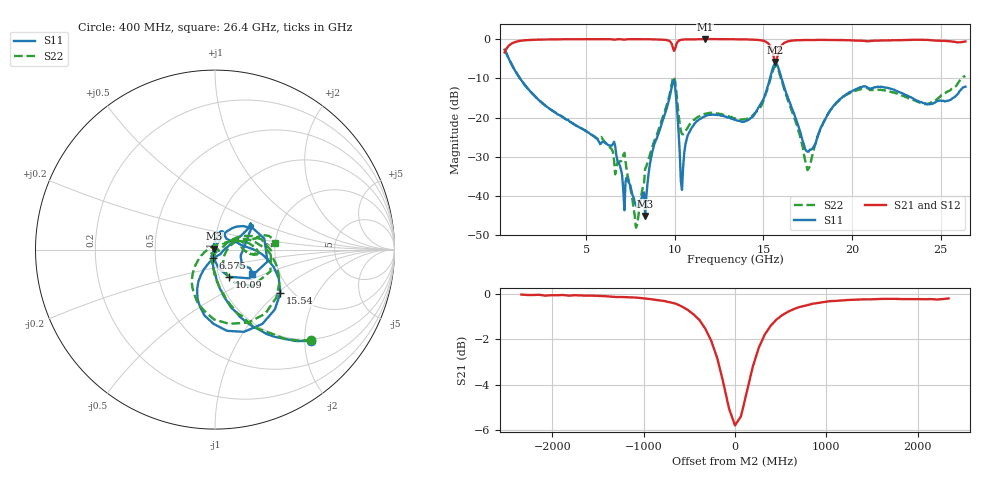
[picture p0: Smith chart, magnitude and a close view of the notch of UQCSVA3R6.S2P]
!  Part Number  UQCSVA3R6  Mounting Orientation: Horizontal
!  Description: Ultra Low ESR Microwave capacitors
!  Application: Coupling, Bypass, Tuning, DC Block
!  Filters, Matching
# GHZ S DB R 50
! Freq  |S11|  S11 Ph  |S21|  S21 Ph  |S12|  S12 Ph  |S22|  S22 Ph
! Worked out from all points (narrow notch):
!   401 points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, 400 MHz to 26.4 GHz, reference 50 ohm
!   highest |S21| = 0.01 dB at 11.71 GHz (marker M1); lowest = -5.8 dB at 15.68 GHz (marker M2)
!   notch at M2: 5.6 dB deep, 396 MHz wide at half that depth
!   lowest |S11| = -45.1 dB at 8.33 GHz (marker M3), VSWR 1.01, Z = 49.7 + j0.443 ohm
!   |S11| at or under -10 dB: 1.266 GHz to 15.37 GHz (14.11 GHz wide, 170 % of centre); 16.02 GHz to end of sweep
!   |S22| runs from -48.1 to -2.6 dB; largest |S21 - S12| = 0.013
!   S11 on the Smith chart (normalised r, x): 400 MHz: 0.96, -2.13; 6.575 GHz: 0.97, -0.09; 10.09 GHz: 1.11, -0.35; 15.54 GHz: 1.75, -1.04; 26.4 GHz: 1.44, -0.42
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0.4  -2.66 -43.7  -3.41 46.2  -3.42 46.1  -2.64 -43.3
1.44  -11.06 -78.1  -0.35 11.6  -0.37 11.5  -11.13 -77.7
4.755  -22.77 -98.1  -0.02 -12.3  -0.04 -12.4  -22.85 -103.3
6.575  -26.18 -103.7  -0.13 -21.1  -0.14 -21.2  -30.87 -133.6
7.16  -43.66 -56.0  -0.15 -23.1  -0.15 -23.2  -29.01 -114.6
7.81  -42.40 -38.8  -0.01 -26.1  -0.01 -26.1  -48.10 -65.2
8.33  -45.14 126.3  -0.01 -28.7  -0.02 -28.8  -33.13 -19.6
9.11  -23.74 64.4  -0.09 -33.0  -0.11 -33.1  -22.77 28.7
9.89  -11.01 12.6  -2.04 -43.0  -2.02 -42.6  -10.11 -0.8
10.085  -15.36 -62.6  -1.42 -24.1  -1.42 -24.6  -13.26 -58.4
10.41  -38.47 145.9  -0.13 -31.5  -0.16 -31.8  -24.24 -31.5
11.71  -19.70 73.4  0.01 -40.7  0.00 -41.0  -19.05 20.4
13.4  -20.56 52.5  -0.05 -49.8  -0.07 -49.9  -20.27 26.3
14.505  -19.18 24.5  -0.15 -57.1  -0.17 -57.2  -18.95 28.9
15.545  -7.19 -33.6  -3.88 -73.3  -3.86 -73.2  -7.94 -25.9
15.675  -6.18 -57.5  -5.80 -58.3  -5.74 -58.3  -6.86 -51.9
16.13  -11.55 -112.0  -1.13 -43.5  -1.15 -43.9  -12.12 -120.4
17.43  -28.55 -71.6  -0.22 -58.2  -0.26 -58.4  -32.13 145.3
17.755  -28.00 -28.7  -0.24 -59.8  -0.26 -60.1  -29.76 60.5
19.38  -15.14 29.1  -0.26 -68.3  -0.27 -68.6  -15.28 14.4
22.11  -12.55 31.3  -0.33 -80.7  -0.35 -80.9  -13.41 -7.0
26.4  -12.15 -33.9  -0.59 -101.7  -0.63 -102.4  -9.39 6.5
